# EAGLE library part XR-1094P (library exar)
EQUALIZER DISPLAY/FILTER/MULTIPLEXER
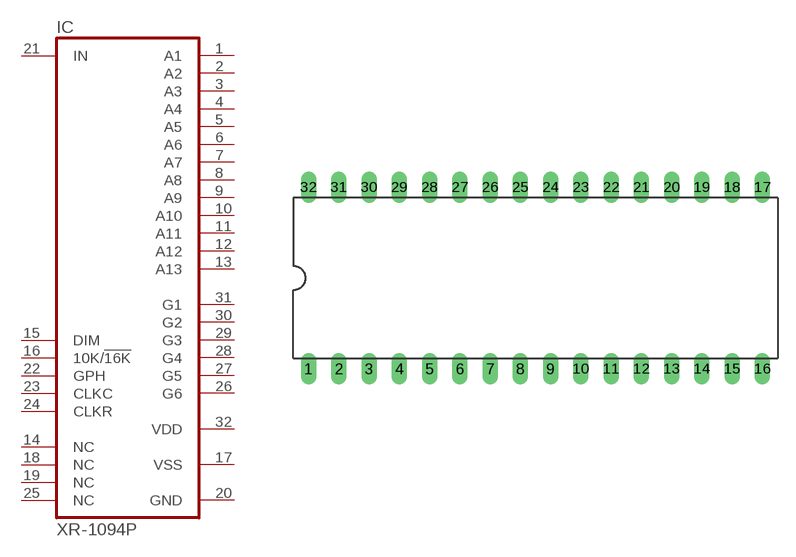
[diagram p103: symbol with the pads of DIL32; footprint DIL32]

Designator prefix IC

## XR-1094P (OC_FARNELL: unknown; OC_NEWARK: unknown)  [DIL32]
1  A1  out
2  A2  out
3  A3  out
4  A4  out
5  A5  out
6  A6  out
7  A7  out
8  A8  out
9  A9  out
10  A10  out
11  A11  out
12  A12  out
13  A13  out
14  NC  nc
15  DIM  in
16  10K/!16K  in
17  VSS  pwr
18  NC  nc
19  NC  nc
20  GND  pwr
21  IN  in
22  GPH  in
23  CLKC  in
24  CLKR  in
25  NC  nc
26  G6  out
27  G5  out
28  G4  out
29  G3  out
30  G2  out
31  G1  out
32  VDD  pwr

## Footprint DIL32 (pad centres in mm)
Dual In Line Package
drill 0.813 long: 1 -19.05,-7.62; 2 -16.51,-7.62; 3 -13.97,-7.62; 4 -11.43,-7.62; 5 -8.89,-7.62; 6 -6.35,-7.62; 7 -3.81,-7.62; 8 -1.27,-7.62; 9 1.27,-7.62; 10 3.81,-7.62; 11 6.35,-7.62; 12 8.89,-7.62; 13 11.43,-7.62; 14 13.97,-7.62; 15 16.51,-7.62; 16 19.05,-7.62; 17 19.05,7.62; 18 16.51,7.62; 19 13.97,7.62; 20 11.43,7.62; 21 8.89,7.62; 22 6.35,7.62; 23 3.81,7.62; 24 1.27,7.62; 25 -1.27,7.62; 26 -3.81,7.62; 27 -6.35,7.62; 28 -8.89,7.62; 29 -11.43,7.62; 30 -13.97,7.62; 31 -16.51,7.62; 32 -19.05,7.62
